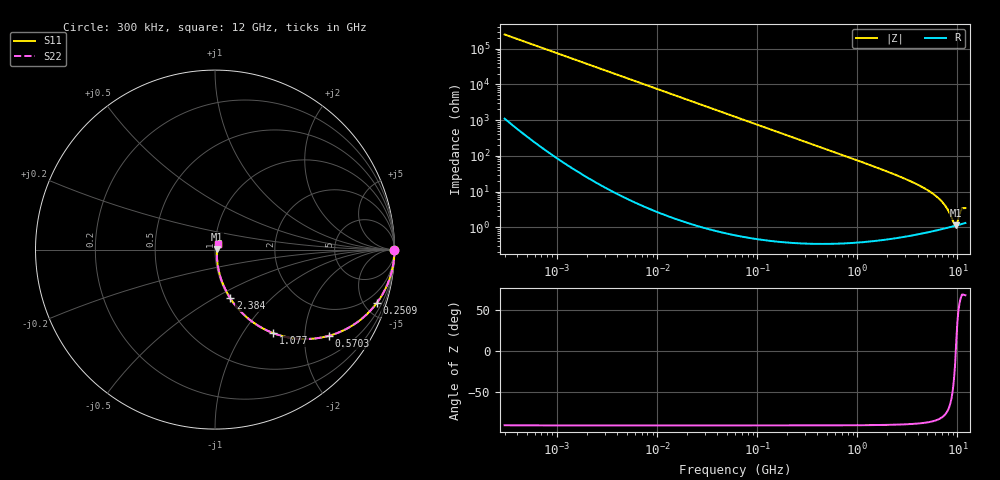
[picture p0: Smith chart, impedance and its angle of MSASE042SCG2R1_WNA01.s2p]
! MSASE042SCG2R1_WNA01  S-PARAMETER MODEL  ( General Type )
! Model Generated by TAIYO YUDEN Corporation (http://www.ty-top.com)
! Version 1.0
! TAIYO YUDEN Control No. 130801
! Copyright(c) 2013 TAIYO YUDEN CO.,LTD. All Rights Reserved.
! Product Description (link to TY-COMPAS)
! https://ds.yuden.co.jp/TYCOMPAS/or/detail?pn=MSASE042SCG2R1AWNA01&u=M
! Products Name : Multilayer Ceramic Capacitors
! Characteristics :
!  Capacitance : 2.1 pF , Rated Voltage : 16V , TCC : CG / C0G
!  Case Size : 0.4 x 0.2 / 0.016 x 0.008 [mm/inch] , Thickness : 0.2 / 0.008 [mm/inch]
!  (Conditions: Temperature = 25 degC , DC Bias Current/Voltage = 0A / 0V)
! External Node Assignments :
!  1  o---| |---o  2
! GND o---------o GND
! Frequency Range : 0.3MHz  -  12000MHz  [ 401 STEP ]
# MHz S RI R 50
! Freq[MHz].  S11 Real  S11 Imag  S21 Real  S21 Imag  S12 Real  S12 Imag  S22 Real  S22 Imag
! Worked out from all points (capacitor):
!   401 points, 300 kHz to 12 GHz, reference 50 ohm
!   read as one part in series: C = 2.11 pF near 316.3 kHz
!   lowest |Z| = 1.13 ohm at 9.708 GHz (marker M1)
!   series resonance near 9.619 GHz, so ESL is about 130 pH
!   S11 on the Smith chart (normalised r, x): 300 kHz: open; 250.9 MHz: 1.01, -6.01; 570.3 MHz: 1.01, -2.63; 1.077 GHz: 1.01, -1.38; 2.384 GHz: 1.01, -0.59; 12 GHz: 1.03, +0.06
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0.3  1 -0.000398  1.9e-06 0.000398  1.9e-06 0.000398  1 -0.000398
1.769972  1 -0.00235  7.2e-06 0.00235  7.2e-06 0.00235  1 -0.00235
10.44266  0.9998 -0.0139  0.000197 0.0139  0.000197 0.0139  0.9998 -0.0139
60  0.9937 -0.0791  0.00633 0.0791  0.00633 0.0791  0.9937 -0.0791
125.9782  0.9727 -0.1626  0.0273 0.1626  0.0273 0.1626  0.9727 -0.1626
250.8588  0.8999 -0.2996  0.1001 0.2996  0.1001 0.2996  0.8999 -0.2996
353.9943  0.8185 -0.3846  0.1815 0.3846  0.1815 0.3846  0.8185 -0.3846
570.2811  0.634 -0.4804  0.366 0.4804  0.366 0.4804  0.634 -0.4804
783.7017  0.4773 -0.4976  0.5227 0.4976  0.5227 0.4976  0.4773 -0.4976
1076.992  0.3242 -0.4654  0.6758 0.4654  0.6758 0.4654  0.3242 -0.4654
1480.043  0.2003 -0.3961  0.7997 0.3961  0.7997 0.3961  0.2003 -0.3961
2088.533  0.1091 -0.3051  0.8909 0.3051  0.8909 0.3051  0.1091 -0.3051
2384.334  0.0848 -0.2704  0.9152 0.2704  0.9152 0.2704  0.0848 -0.2704
4050.141  0.0289 -0.1481  0.9711 0.1481  0.9711 0.1481  0.0289 -0.1481
5868.704  0.0142 -0.0793  0.9858 0.0793  0.9858 0.0793  0.0142 -0.0793
7254.098  0.011 -0.0445  0.989 0.0445  0.989 0.0445  0.011 -0.0445
8064.993  0.0104 -0.0278  0.9896 0.0278  0.9896 0.0278  0.0104 -0.0278
9207.246  0.0107 -0.00741  0.9893 0.00741  0.9893 0.00741  0.0107 -0.00741
9708.23  0.0111 0.00187  0.9889 -0.00187  0.9889 -0.00187  0.0111 0.00187
9968.853  0.0113 0.00752  0.9887 -0.00752  0.9887 -0.00752  0.0113 0.00752
11083.22  0.0131 0.0304  0.9869 -0.0304  0.9869 -0.0304  0.0131 0.0304
12000  0.014 0.0309  0.986 -0.0309  0.986 -0.0309  0.014 0.0309
